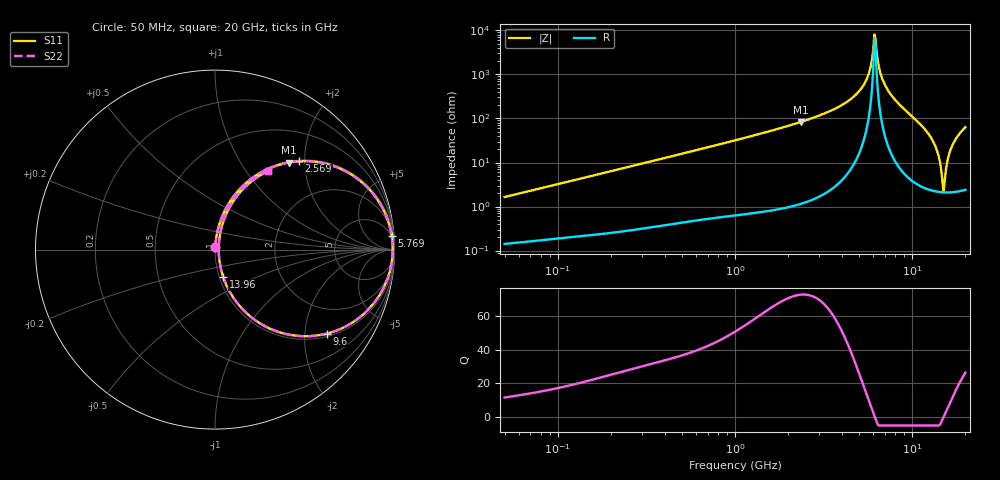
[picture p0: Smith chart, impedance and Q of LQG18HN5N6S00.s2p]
!Murata Part Number: LQG18HN5N6S00
!These Parameters are Measured in Series Mode Connection
!  o--[Z]--o
!Port1  Port2
!  o-------o
!Freq. Start=50[MHz] Stop=20[GHz], 401[Steps]
# Hz S RI R 50
!Freq.(Hz) S11(Real) S11(Imag) S21(Real) S21(Imag) S12(Real) S12(Imag) S22(Real) S22(Imag)
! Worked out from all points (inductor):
!   401 points, 50 MHz to 20 GHz, reference 50 ohm
!   read as one part in series: L = 5.18 nH near 51.52 MHz
!   highest Q = 72.7 at 2.349 GHz (marker M1), where L = 5.64 nH
!   self-resonance near 6.125 GHz
!   S11 on the Smith chart (normalised r, x): 50 MHz: 1.00, +0.03; 2.569 GHz: 1.03, +1.87; 5.769 GHz: 4, +25; 9.6 GHz: 1.09, -2.59; 13.96 GHz: 1.04, -0.33; 20 GHz: 1.05, +1.27
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5e7  0.00168 0.0163  0.9983 -0.0163  0.9983 -0.0163  0.00168 0.0163
1.364002e8  0.00401 0.0434  0.996 -0.0434  0.996 -0.0434  0.00401 0.0434
3.721004e8  0.0171 0.1152  0.9829 -0.1152  0.9829 -0.1152  0.0171 0.1152
1e9  0.0965 0.2855  0.9035 -0.2855  0.9035 -0.2855  0.0965 0.2855
2.348516e9  0.4101 0.485  0.5899 -0.485  0.5899 -0.485  0.4101 0.485
2.569357e9  0.4681 0.4921  0.5319 -0.4921  0.5319 -0.4921  0.4681 0.4921
2.728004e9  0.5092 0.493  0.4908 -0.493  0.4908 -0.493  0.5092 0.493
4.608136e9  0.8913 0.2979  0.1087 -0.2979  0.1087 -0.2979  0.8913 0.2979
5.273168e9  0.9588 0.1749  0.0412 -0.1749  0.0412 -0.1749  0.9588 0.1749
5.769027e9  0.9843 0.0774  0.0157 -0.0774  0.0157 -0.0774  0.9843 0.0774
6.034176e9  0.9894 0.0249  0.0106 -0.0249  0.0106 -0.0249  0.9894 0.0249
6.217679e9  0.9897 -0.0112  0.0103 0.0112  0.0103 0.0112  0.9897 -0.0112
6.701223e9  0.9779 -0.1041  0.0221 0.1041  0.0221 0.1041  0.9779 -0.1041
7.442007e9  0.9277 -0.2347  0.0723 0.2347  0.0723 0.2347  0.9277 -0.2347
9.600142e9  0.6234 -0.468  0.3766 0.468  0.3766 0.468  0.6234 -0.468
1.220001e10  0.2011 -0.3759  0.7989 0.3759  0.7989 0.3759  0.2011 -0.3759
1.396067e10  0.0457 -0.1528  0.9543 0.1528  0.9543 0.1528  0.0457 -0.1528
1.460232e10  0.0248 -0.0626  0.9752 0.0626  0.9752 0.0626  0.0248 -0.0626
1.504638e10  0.0206 -0.00116  0.9794 0.00116  0.9794 0.00116  0.0206 -0.00116
1.621653e10  0.0435 0.1483  0.9565 -0.1483  0.9565 -0.1483  0.0435 0.1483
1.696185e10  0.0782 0.2301  0.9218 -0.2301  0.9218 -0.2301  0.0782 0.2301
2e10  0.295 0.4375  0.705 -0.4375  0.705 -0.4375  0.295 0.4375
